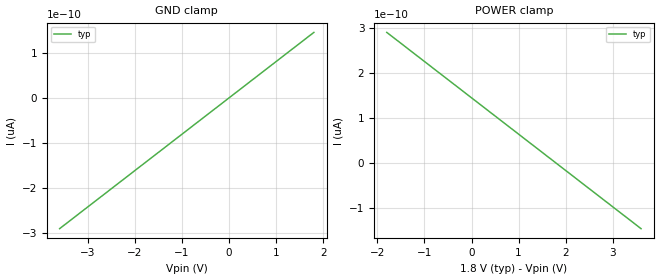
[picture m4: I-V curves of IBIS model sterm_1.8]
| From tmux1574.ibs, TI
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| sterm_1.8
[Model]   sterm_1.8
Model_type   Terminator
|   typ   min   max
C_comp   4.014581e-12   NA   NA
[Voltage Range]   1.8   NA   NA
[Temperature Range]   27   NA   NA
[Power Clamp Reference]   1.8   NA   NA
[GND Clamp Reference]   0   NA   NA
[GND Clamp]
|   Voltage   I(typ)   I(min)   I(max)
-3.6V     0A         NA         NA
-3.545V   0A         NA         NA
600mV     0A         NA         NA
1.8V      0A         NA         NA
[POWER Clamp]
|   Voltage   I(typ)   I(min)   I(max)
-1.8V     0A         NA         NA
1.2V      0A         NA         NA
3.055V    0A         NA         NA
3.6V      0A         NA         NA
